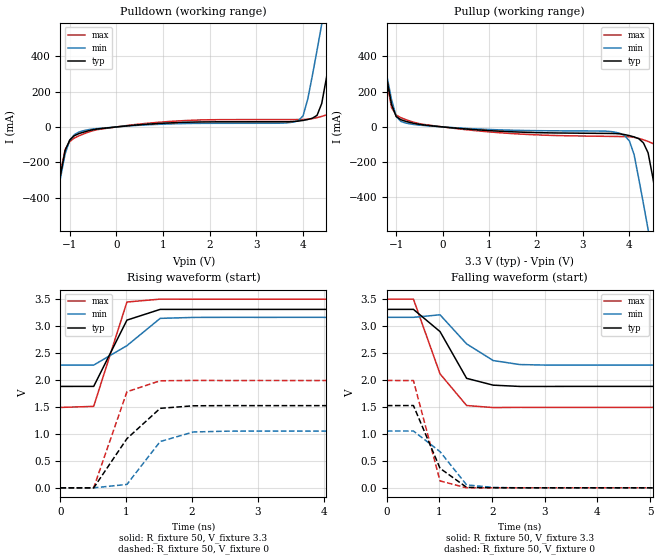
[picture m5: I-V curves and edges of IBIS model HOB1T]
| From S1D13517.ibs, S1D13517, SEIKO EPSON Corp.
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[Model]   HOB1T
Model_type Output
Polarity Non-Inverting
C_comp   5p   4p   6p
[Temperature Range] 50   100   0
[Voltage Range]   3.3   3.0   3.6
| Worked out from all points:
|   slope of the pulldown table from 0 to 0.495 V, typ, clamps not added: 40.5 ohm
|   slope of the pullup table from 0 to 0.495 V, typ, clamps not added: 42.6 ohm
|   falling waveform, R_fixture 50, V_fixture 3.3: 20-80 % time 580ps typ, 648ps min, 548ps max; typ from 3.3 V to 1.88 V
|   falling waveform, R_fixture 50, V_fixture 0: 20-80 % time 454ps typ, 603ps min, 324ps max; typ from 1.52 V to 0 V
|   rising waveform, R_fixture 50, V_fixture 3.3: 20-80 % time 352ps typ, 605ps min, 314ps max; typ from 1.88 V to 3.3 V
|   rising waveform, R_fixture 50, V_fixture 0: 20-80 % time 612ps typ, 401ps min, 339ps max; typ from 0 V to 1.52 V
[Pullup]
-3.3V     3.687A     3.389A     4.049A
-1.4V     592.9mA    581.8mA    608.6mA
-1.1V     128mA      156.1mA    110.8mA
-900mV    41.08mA    31.54mA    52.69mA
900mV     -19.27mA   -13.49mA   -25.91mA
3.6V      -36.94mA   -26.11mA   -53.67mA
3.9V      -43.64mA   -50.13mA   -54.8mA
4.1V      -56.52mA   -157mA     -58.91mA
4.4V      -146.8mA   -581mA     -82.35mA
4.7V      -601.7mA   -1.02A     -154.8mA
5V        -1.087A    -1.46A     -634.1mA
6.6V      -3.692A    -3.821A    -3.546A
[Pulldown]
-3.3V     -3.684A    -3.376A    -4.079A
-1.4V     -591.9mA   -578.3mA   -616.1mA
-1.1V     -133.3mA   -152.9mA   -128.3mA
-800mV    -37.62mA   -28.47mA   -50.17mA
3.9V      33.09mA    35.69mA    41.78mA
4.1V      42.11mA    157.5mA    43.49mA
4.3V      65.66mA    435mA      52.54mA
4.4V      132.3mA    581.6mA    59.65mA
4.5V      276.6mA    728.4mA    68.34mA
4.7V      595.1mA    1.022A     121.9mA
5V        1.082A     1.464A     615.3mA
6.6V      3.687A     3.828A     3.513A
[Falling Waveform]
R_fixture=50
V_fixture=3.3
0s        3.3V       3.153V     3.488V
505.1ps   3.3V       3.153V     3.489V
1.01ns    2.889V     3.2V       2.108V
1.515ns   2.024V     2.661V     1.522V
2.02ns    1.898V     2.353V     1.484V
2.525ns   1.875V     2.279V     1.488V
3.03ns    1.874V     2.269V     1.487V
50ns      1.876V     2.269V     1.487V
[Falling Waveform]
R_fixture=50
V_fixture=0
0s        1.52V      1.05V      1.985V
505.1ps   1.521V     1.05V      1.983V
1.01ns    360.8mV    669.4mV    127mV
1.515ns   7.943mV    53.36mV    -1.317mV
2.02ns    873.3uV    6.645mV    -79.92uV
2.525ns   -40.37uV   -494.4uV   21.75uV
50ns      10.04uV    55.87uV    4.735uV
[Rising Waveform]
R_fixture=50
V_fixture=3.3
0s        1.876V     2.269V     1.487V
505.1ps   1.876V     2.27V      1.507V
1.01ns    3.102V     2.63V      3.436V
1.515ns   3.3V       3.134V     3.49V
2.02ns    3.3V       3.151V     3.488V
2.525ns   3.3V       3.153V     3.489V
50ns      3.3V       3.153V     3.488V
[Rising Waveform]
R_fixture=50
V_fixture=0
0s        0V         0V         0V
505.1ps   2.445uV    -4.142uV   1.802mV
1.01ns    910.2mV    63.71mV    1.777V
1.515ns   1.471V     856.6mV    1.98V
2.02ns    1.517V     1.033V     1.986V
2.525ns   1.521V     1.048V     1.985V
50ns      1.52V      1.05V      1.985V
[Ramp]
R_load=50
dV/dt_r   9.122E-1/3.201E-10   6.298E-1/3.987E-10   1.191E+0/2.587E-10
dV/dt_f   8.547E-1/4.183E-10   6.141E-1/4.864E-10   1.153E+0/3.509E-10
|[End   HOB1T
